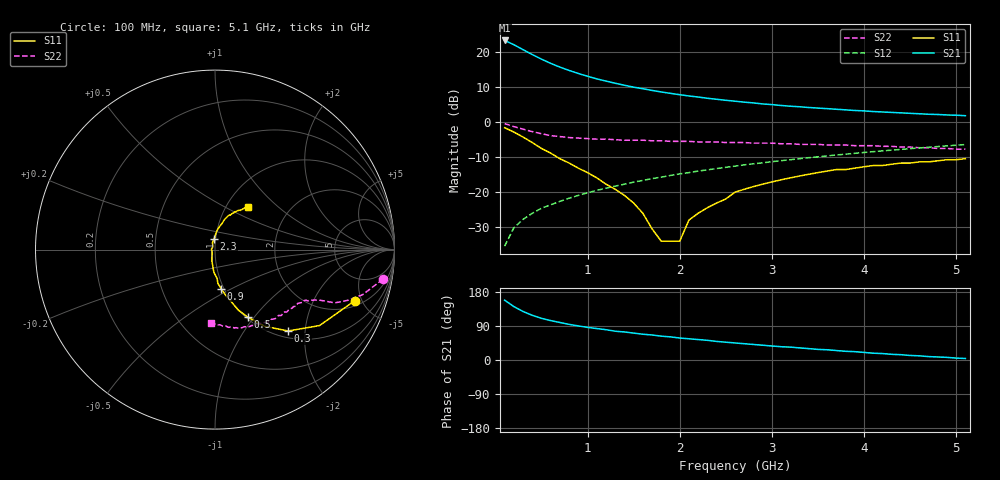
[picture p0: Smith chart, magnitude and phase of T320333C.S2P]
!AT-32033
!S PARAMETERS at Vce=2.7V  Ic=5mA.  LAST UPDATED 01-05-95
# ghz s ma r 50
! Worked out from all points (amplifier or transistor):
!   51 points, 100 MHz to 5.1 GHz, reference 50 ohm
!   highest |S21| = 23.2 dB at 100 MHz (marker M1)
!   |S21| within 3 dB of that: start of sweep to 326.9 MHz
!   unconditionally stable (mu >= 1): 1.31 GHz to 2.583 GHz
!   at 900 MHz: K = 0.93, MSG = 17.4 dB, |S12| = -20.9 dB
!   at 2.6 GHz: K = 1.00, MSG = 9.3 dB, |S12| = -12.6 dB
!   at 5.1 GHz: K = 0.91, MSG = 4.1 dB, |S12| = -6.4 dB
!   S11 on the Smith chart (normalised r, x): 100 MHz: 2.41, -4.40; 300 MHz: 1.13, -1.63; 500 MHz: 1.02, -0.93; 900 MHz: 0.97, -0.44; 2.3 GHz: 0.98, +0.12; 5.1 GHz: 1.26, +0.66
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0.1  0.83 -20.0  14.53 158.0  0.017 79.0  0.95 -10.0
0.2  0.72 -36.0  12.65 141.0  0.031 72.0  0.86 -17.0
0.3  0.61 -48.0  10.74 128.0  0.041 68.0  0.79 -21.0
0.4  0.51 -57.0  9.15 118.0  0.05 67.0  0.73 -24.0
0.5  0.42 -64.0  7.87 110.0  0.059 66.0  0.68 -25.0
0.6  0.36 -69.0  6.85 104.0  0.066 65.0  0.64 -26.0
0.7  0.3 -73.0  6.06 99.0  0.074 65.0  0.62 -27.0
0.8  0.26 -77.0  5.43 94.0  0.082 66.0  0.6 -28.0
0.9  0.22 -81.0  4.91 90.0  0.09 66.0  0.59 -29.0
1  0.19 -85.0  4.49 86.0  0.098 65.0  0.58 -29.0
1.1  0.16 -86.0  4.12 83.0  0.106 65.0  0.57 -30.0
1.3  0.11 -95.0  3.57 76.0  0.122 65.0  0.56 -32.0
1.6  0.05 -110.0  2.98 68.0  0.147 64.0  0.55 -35.0
1.8  0.02 -145.0  2.68 63.0  0.164 63.0  0.54 -37.0
2  0.02 126.0  2.45 58.0  0.182 62.0  0.53 -40.0
2.1  0.04 111.0  2.35 56.0  0.19 61.0  0.53 -41.0
2.3  0.06 96.0  2.18 52.0  0.208 59.0  0.52 -44.0
2.6  0.1 85.0  1.98 45.0  0.235 57.0  0.51 -48.0
3.1  0.15 75.0  1.72 35.0  0.281 53.0  0.49 -56.0
3.5  0.19 70.0  1.58 28.0  0.319 49.0  0.48 -62.0
4.3  0.25 60.0  1.37 15.0  0.397 41.0  0.45 -76.0
5.1  0.3 52.0  1.23 4.0  0.477 32.0  0.41 -93.0
